TYPE LstTCPUnit :
STRUCT
	TCP_UnitName: STRING;
	TCP_RFPower: INT;
	TCP_TuneCapPreset: INT;
	TCP_LoadCapPreset: INT;
	TCP_AutoTuneCapPreset: INT;
	TCP_AutoLoadCapPreset: INT;
	TCP_MaxReflectedPower: INT;
	TCP_EnableRamp: BOOL;
	TCP_TargetRFPower: INT;
END_STRUCT
END_TYPE
